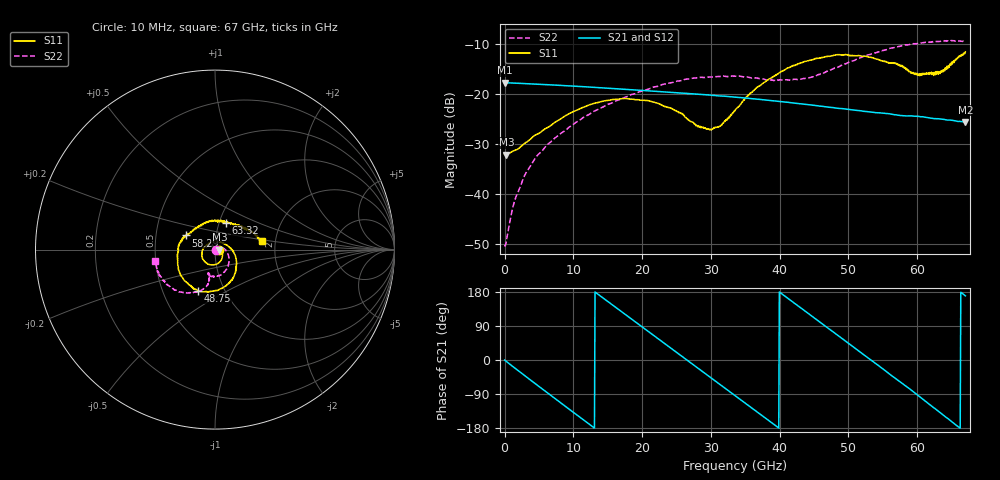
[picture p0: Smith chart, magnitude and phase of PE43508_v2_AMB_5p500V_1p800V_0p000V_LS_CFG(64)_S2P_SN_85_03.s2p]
!Keysight Technologies,N5227A,US51270237,A.10.43.00
!Date: Wednesday, August 22, 2018 17:13:17
!Correction: S11(Full 2 Port(1,3))
!S31(Full 2 Port(1,3))
!S13(Full 2 Port(1,3))
!S33(Full 2 Port(1,3))
!S2P File: Measurements: S11, S31, S13, S33:
# Hz S  dB  R 50
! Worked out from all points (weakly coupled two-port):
!   801 points, 10 MHz to 67 GHz, reference 50 ohm
!   highest |S21| = -17.72 dB at 10 MHz (marker M1); lowest = -25.6 dB at 67 GHz (marker M2)
!   lowest |S11| = -32.1 dB at 261.2 MHz (marker M3), VSWR 1.05, Z = 52.5 - j0.00317 ohm
!   |S11| at or under -10 dB: start of sweep to end of sweep
!   |S22| runs from -50.5 to -9.3 dB; largest |S21 - S12| = 0.00068
!   S11 on the Smith chart (normalised r, x): 10 MHz: 1.05, -0.00; 48.75 GHz: 0.75, -0.37; 58.29 GHz: 0.71, +0.12; 63.32 GHz: 1.08, +0.33; 67 GHz: 1.69, +0.17
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1e7  -32.06 -1.0  -17.72 -0.2  -17.72 -0.2  -50.35 -2.7
2.612125e8  -32.14 -0.1  -17.75 -3.9  -17.76 -3.9  -49.58 23.5
1.517275e9  -31.29 -1.8  -17.83 -21.6  -17.83 -21.6  -41.20 49.4
3.443238e9  -29.42 -9.8  -17.95 -48.4  -17.96 -48.4  -35.12 43.7
6.206575e9  -26.76 -26.6  -18.13 -86.3  -18.13 -86.3  -30.20 30.6
1.123082e10  -22.77 -67.1  -18.52 -154.7  -18.52 -154.7  -24.93 -0.5
1.74274e10  -20.91 -115.6  -19.05 121.8  -19.05 121.9  -20.69 -32.3
2.236791e10  -21.92 -155.2  -19.50 55.6  -19.50 55.6  -18.39 -55.1
2.605236e10  -24.31 168.5  -19.84 6.4  -19.83 6.3  -17.14 -71.1
2.797832e10  -26.33 134.3  -20.03 -19.5  -20.03 -19.6  -16.77 -78.2
2.973681e10  -27.10 98.5  -20.21 -43.1  -20.21 -43.1  -16.57 -84.9
3.132782e10  -26.45 63.1  -20.38 -64.4  -20.39 -64.3  -16.49 -90.7
3.3505e10  -23.35 22.7  -20.63 -93.8  -20.64 -93.9  -16.43 -97.6
3.836178e10  -17.13 -30.6  -21.26 -159.1  -21.27 -159.0  -17.21 -105.8
4.472582e10  -13.16 -82.1  -22.21 115.1  -22.20 115.3  -16.62 -101.2
4.874522e10  -12.15 -112.1  -22.90 61.2  -22.89 61.1  -14.44 -101.6
5.251341e10  -12.46 -143.1  -23.50 10.0  -23.47 10.0  -12.30 -109.3
5.586291e10  -13.83 -177.0  -23.94 -35.5  -23.92 -35.9  -10.92 -121.6
5.82913e10  -14.84 154.3  -24.39 -68.2  -24.39 -68.5  -10.18 -131.0
6.004979e10  -15.91 125.1  -24.47 -92.5  -24.48 -92.9  -9.90 -138.5
6.331555e10  -15.90 67.6  -25.00 -138.7  -25.04 -139.2  -9.46 -153.0
6.7e10  -11.56 10.2  -25.59 169.2  -25.67 169.2  -9.38 -169.1
